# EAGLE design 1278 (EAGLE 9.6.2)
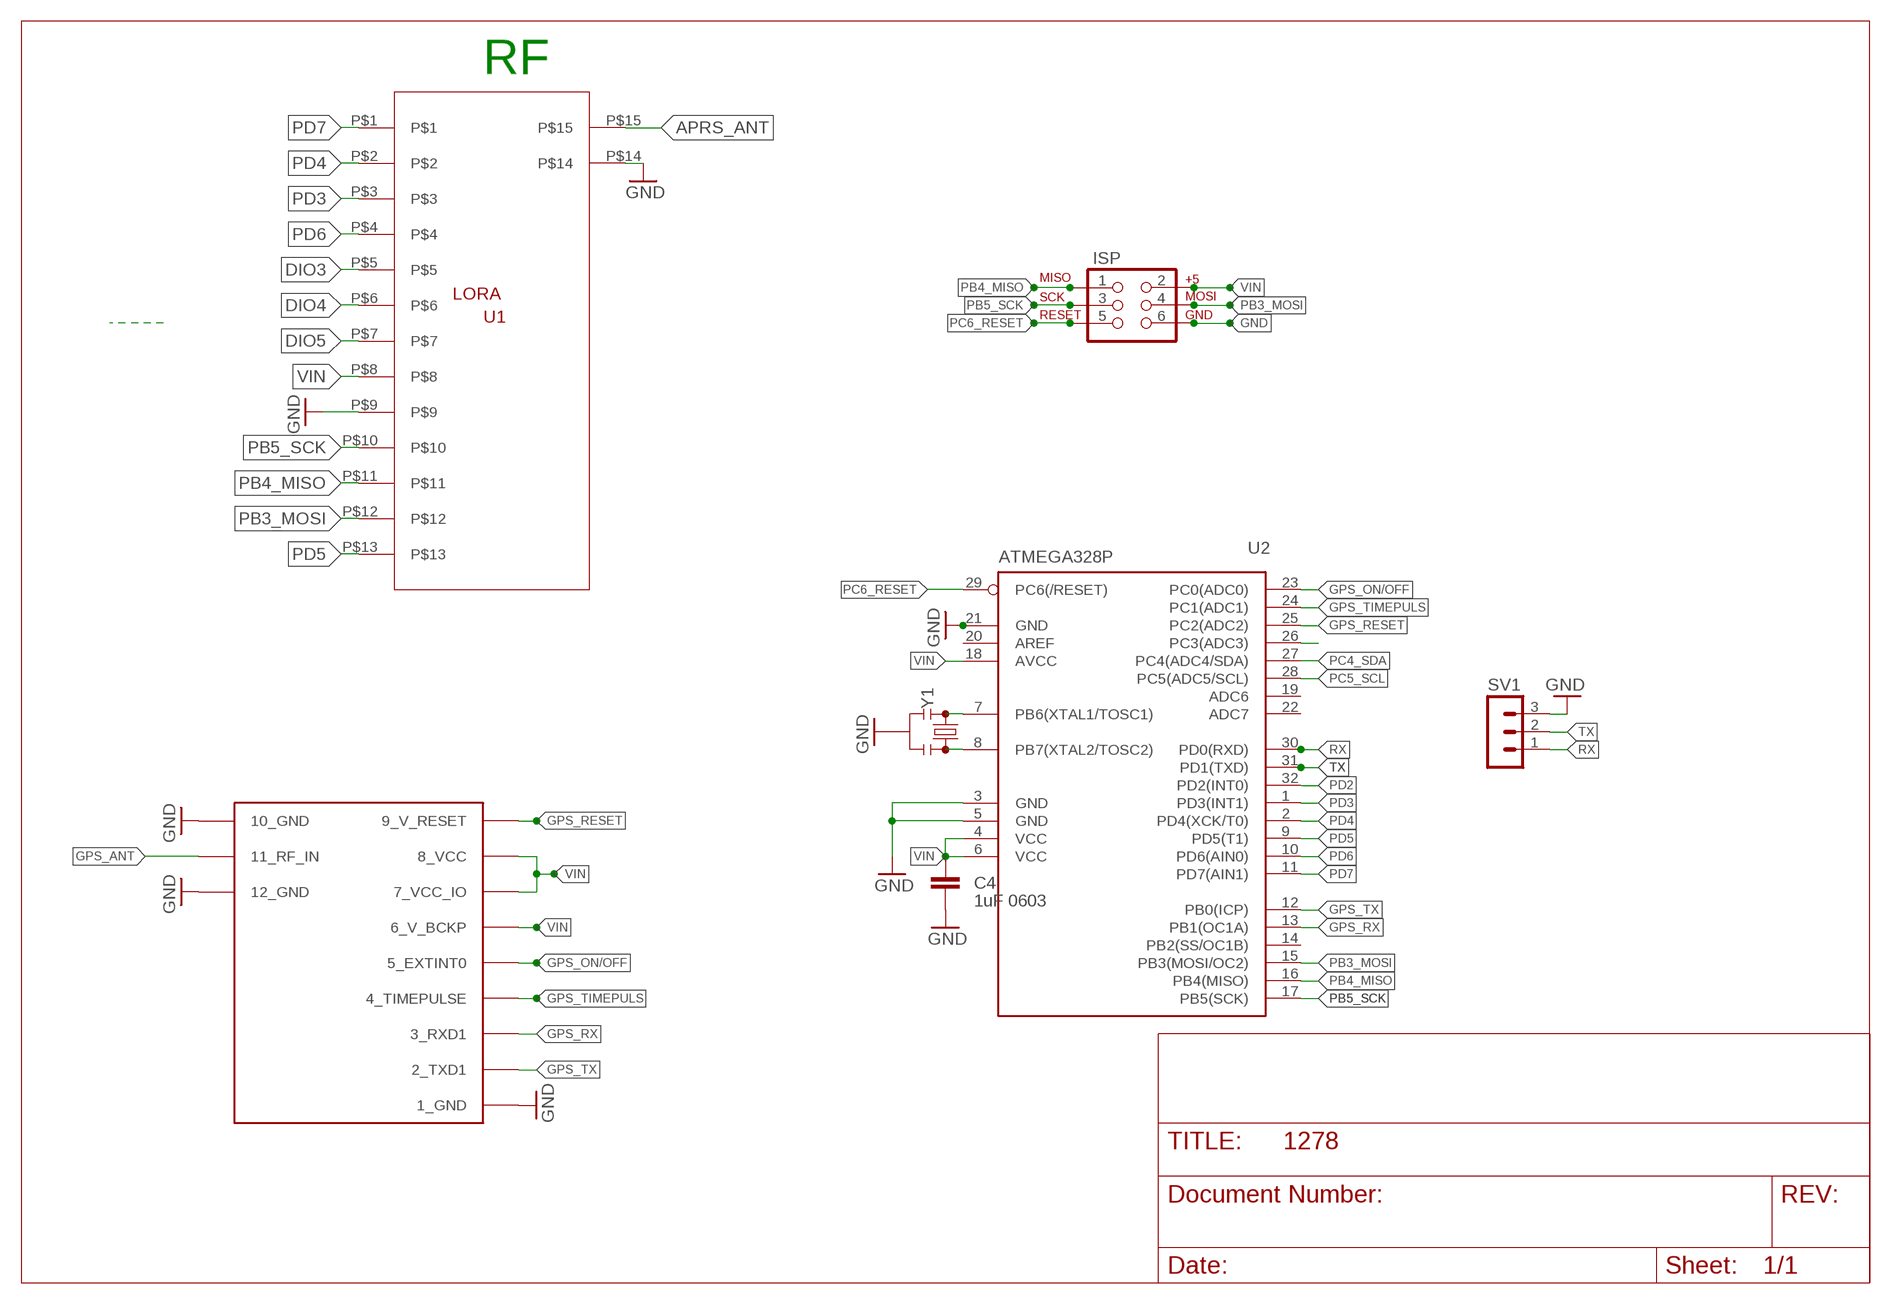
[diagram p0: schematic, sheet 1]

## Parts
C4  1uF 0603  C-EUC0603K  [C0603K]
ISP  AVR_SPI_PRG_6PTH  [2X3]
SV1  MA03-1  [MA03-1]
U1  LORA  [LORA_DRF]
U2  ATMEGA328P  MEGA8-AI  [TQFP32-08]
U$2  UBLOX_MAX  [UBLOX_MAX]
Y1  RESONATORSMD-4.5X2.0  [RESONATOR-SMD-4.5X2.0]

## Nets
APRS_ANT: U1.P$15
DIO3: U1.P$5
DIO4: U1.P$6
DIO5: U1.P$7
GND: C4.2 ISP.6 SV1.3 U1.P$9 U1.P$14 U2.3(GND) U2.5(GND) U2.21(GND) U$2.1_GND U$2.10_GND U$2.12_GND Y1.2
GPS_ANT: U$2.11_RF_IN
GPS_ON/OFF: U2.23(PC0(ADC0)) U$2.5_EXTINT0
GPS_RESET: U2.25(PC2(ADC2)) U$2.9_V_RESET
GPS_RX: U2.13(PB1(OC1A)) U$2.3_RXD1
GPS_TIMEPULS: U2.24(PC1(ADC1)) U$2.4_TIMEPULSE
GPS_TX: U2.12(PB0(ICP)) U$2.2_TXD1
N$1: U2.8(PB7(XTAL2/TOSC2)) Y1.3
N$2: U2.7(PB6(XTAL1/TOSC1)) Y1.1
N$10: U2.26(PC3(ADC3))
PB3_MOSI: ISP.4 U1.P$12 U2.15(PB3(MOSI/OC2))
PB4_MISO: ISP.1 U1.P$11 U2.16(PB4(MISO))
PB5_SCK: ISP.3 U1.P$10 U2.17(PB5(SCK))
PC4_SDA: U2.27(PC4(ADC4/SDA))
PC5_SCL: U2.28(PC5(ADC5/SCL))
PC6_RESET: ISP.5 U2.29(PC6(/RESET))
PD2: U2.32(PD2(INT0))
PD3: U1.P$3 U2.1(PD3(INT1))
PD4: U1.P$2 U2.2(PD4(XCK/T0))
PD5: U1.P$13 U2.9(PD5(T1))
PD6: U1.P$4 U2.10(PD6(AIN0))
PD7: U1.P$1 U2.11(PD7(AIN1))
RX: SV1.1 U2.30(PD0(RXD))
TX: SV1.2 U2.31(PD1(TXD))
VIN: C4.1 ISP.2 U1.P$8 U2.4(VCC) U2.6(VCC) U2.18(AVCC) U$2.6_V_BCKP U$2.7_VCC_IO U$2.8_VCC
Unconnected: U2.14(PB2(SS/OC1B)) U2.19(ADC6) U2.20(AREF) U2.22(ADC7)

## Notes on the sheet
- RF

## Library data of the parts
C4 = rcl:C-EU: CAPACITOR, European symbol; SPICEPREFIX: C
ISP = SparkFun:AVR_SPI_PRG_6: AVR ISP 6 Pin This is the reduced ISP connector for AVR programming. Common on Arduino. This footprint will take up less PCB space and can be used with a 10-pin to 6-pin adapter such as SKU: BOB-08508
SV1 = con-lstb:MA03-1: PIN HEADER; OC_FARNELL: unknown; OC_NEWARK: unknown
U1 = lora:LORA
U2 = atmel:MEGA8: MICROCONTROLLER 8 Kbytes FLASH, 1 kbytes SRAM, 512 bytes EEPROM, USART, 6-channel 10 bit ADC, 2-channel 8 bit ADC Pin compatible with Atmega48, ATMega88, ATMega168 Source: avr.lbr; MPN: ATMEGA8-16AU; OC_FARNELL: 9171371; OC_NEWARK: 73M8863
U$2 = Max gps:UBLOX_MAX: UBLOX MAX
Y1 = SparkFun-Clocks:RESONATOR: Resonators (Generic) Ceramic resonators are clock-generating components, often used to control timing in microcontrollers. They usually have 3 pins: two pins for oscillation, and one pin for ground. Compared to crystals, resonators have worse tolerance, but are usually much cheaper. Plus, they have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

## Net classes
0 default: width 0.152 mm, drill 0.305 mm, clearance 0.152 mm
1 vcc: width 0.152 mm, clearance 0.152 mm

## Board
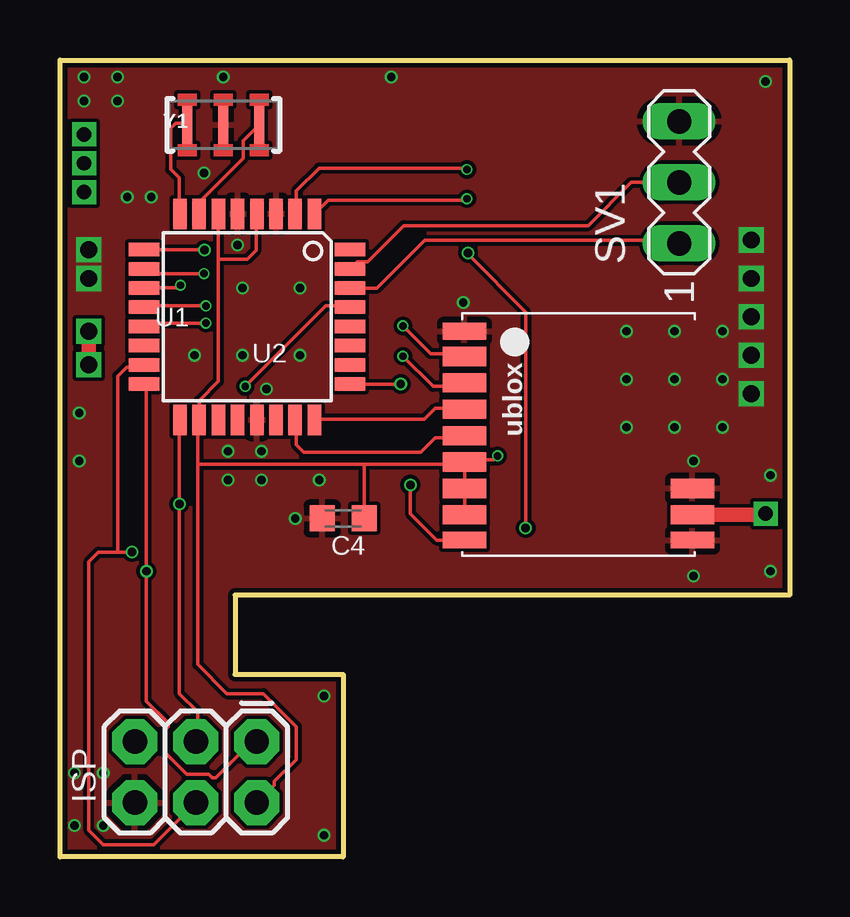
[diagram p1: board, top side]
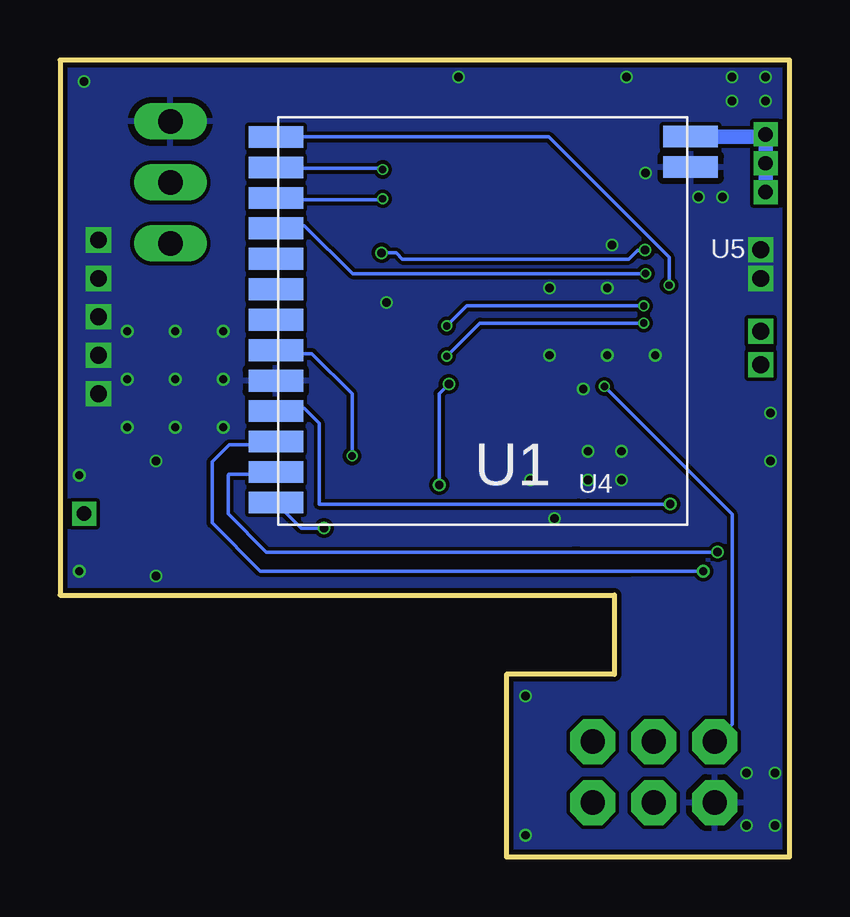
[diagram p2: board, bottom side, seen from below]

Size 30.4 x 33.2 mm. Coordinates in mm from the lower left corner, seen from the top.
Outline: 0,33.2 30.4,33.2 30.4,10.9 7.3,10.9 7.3,7.6 11.8,7.6 11.8,0 0,0 0,33.2
Copper layers (1*16): Top 0.035559375mm / dielectric 1.6mm / Bottom 0.035559375mm
Design rules "jlcpcb2layer *": minimum track width 5mil, minimum drill 12mil, track to track 5mil, track to pad 5mil, pad to pad 5mil, via to via 5mil, smd to smd 5mil, copper to edge 8mil, drill to drill 6mil, minimum pad ring 5mil, minimum via ring 3mil, stop-mask expansion 2.5mil, vias tented up to drill 14mil, thermal gap 10mil

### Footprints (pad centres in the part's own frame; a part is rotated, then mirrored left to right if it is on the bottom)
C0603K = smd 1.05 x 1.08: 1 -0.875,0; 2 0.875,0
2X3 = drill 1.016 pad 1.88 octagon: 1 0,0; 2 0,2.54; 3 2.54,0; 4 2.54,2.54; 5 5.08,0; 6 5.08,2.54
MA03-1 = drill 1.016 long: 1 -2.54,0; 2 0,0; 3 2.54,0
LORA_DRF = smd 2.27 x 0.9: P$1 -8.609,7.497; P$2 -8.609,6.227; P$3 -8.608,4.958; P$4 -8.608,3.688; P$5 -8.609,2.417; P$6 -8.609,1.147; P$7 -8.608,-0.122; P$8 -8.608,-1.392; P$9 -8.61,-2.663; P$10 -8.61,-3.933; P$11 -8.609,-5.202; P$12 -8.609,-6.472; P$13 -8.609,-7.743; P$14 8.673,6.235; P$15 8.675,7.506
TQFP32-08 = smd 1.27 x 0.559: 1 -4.293,2.8; 2 -4.293,2; 3 -4.293,1.2; 4 -4.293,0.4; 5 -4.293,-0.4; 6 -4.293,-1.2; 7 -4.293,-2; 8 -4.293,-2.8; 17 4.293,-2.8; 18 4.293,-2; 19 4.293,-1.2; 20 4.293,-0.4; 21 4.293,0.4; 22 4.293,1.2; 23 4.293,2; 24 4.293,2.8 | smd 0.559 x 1.27: 9 -2.8,-4.293; 10 -2,-4.293; 11 -1.2,-4.293; 12 -0.4,-4.293; 13 0.4,-4.293; 14 1.2,-4.293; 15 2,-4.293; 16 2.8,-4.293; 25 2.8,4.293; 26 2,4.293; 27 1.2,4.293; 28 0.4,4.293; 29 -0.4,4.293; 30 -1.2,4.293; 31 -2,4.293; 32 -2.8,4.293
UBLOX_MAX = smd 1.8 x 0.7: 1_GND 4.95,-4.4; 9_V_RESET 4.95,4.3; 10_GND -4.55,4.3 | smd 1.8 x 0.8: 2_TXD1 4.95,-3.35; 3_RXD1 4.95,-2.25; 4_TIMEPULSE 4.95,-1.15; 5_EXTINT0 4.95,-0.05; 6_V_BCKP 4.95,1.05; 7_VCC_IO 4.95,2.15; 8_VCC 4.95,3.25; 11_RF_IN -4.55,3.25; 12_GND -4.55,2.15
RESONATOR-SMD-4.5X2.0 = smd 0.4 x 1.6: 1 -1.5,0; 2 0,0; 3 1.5,0

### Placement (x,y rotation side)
C4  11.8,14.1 180 top
ISP  8.2,4.8 180 top
SV1  25.8,28.1 90 top
U1  12.8,22.5 0 bottom
U2  7.8,22.5 270 top
U$2  21.8,17.5 180 top
Y1  6.8,30.5 180 top

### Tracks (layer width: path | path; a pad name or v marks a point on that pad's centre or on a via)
APRS_ANT  (via drill 0.6 pad 1)
  Bottom 0.61: U1.P$15 1.09,30.01 v1,30.1 v1,28.9 v1,27.7
GND  (via drill 0.35, 0.7 pad 1)
  Top 0.152: U2.5 7.41,26.76 7.44,26.83
  other vias: 2.8,27.5 13.8,32.5 23.6,19.9 26.4,11.7 7.6,20.9 10.8,15.7 9.8,14.1 0.8,18.5 26.4,16.5 16.8,23.1 10,20.9 8.6,19.5 6.8,32.5 7.4,25.5 6,28.5 3.8,27.5 8.4,16.9 7,16.9 7,15.7 8.4,15.7 7.6,23.7 10,23.7 1.2,24.1 1.2,25.3 28.8,25.7 28.8,24.1 28.8,22.5 28.8,20.9 28.8,19.3 23.6,21.9 25.6,21.9 27.6,21.9 27.6,19.9 25.6,19.9 25.6,17.9 27.6,17.9 23.6,17.9 29.6,15.9 29.6,11.9 5.6,20.9 0.8,16.5 1.8,3.5 11,6.7 11,0.9 1.8,1.3 0.6,3.5 0.6,1.3 29.4,32.3 1,32.5 2.4,32.5 1,31.5 2.4,31.5
  pour Top: -4.59,41.22 49.35,41.22 49.35,-1.89 -4.59,-1.89
  pour Bottom: -4.59,41.22 49.35,41.22 49.35,-1.89 -4.59,-1.89
GPS_ANT  (via drill 0.6 pad 1)
  Top 0.152: 29.35,14.25 v29.4,14.3
  Top 0.61: U$2.11_RF_IN 29.35,14.25
GPS_ON/OFF
  Top 0.152: 16.71,17.46 16.74,17.46 16.84,17.56 | 16.71,17.46 15.64,17.46 15.03,16.86 10.16,16.86 9.85,17.16 9.85,18.07 9.82,18.21 9.85,18.23 U2.23 | 16.71,17.46 U$2.5_EXTINT0
GPS_RESET  (via drill 0.35)
  Top 0.152: U2.25 12.14,19.75 U2.25 v14.2,19.7 | v14.6,15.5 14.6,14.3 15.7,13.2 U$2.9_V_RESET
  Bottom 0.152: v14.2,19.7 14.6,19.3 v14.6,15.5
GPS_RX  (via drill 0.3)
  Top 0.152: v6.08,22.24 3.64,22.24 U2.13 3.6,22.04 3.59,22.04 U2.13 | v14.29,20.86 15.55,19.6 16.7,19.6 | 16.7,19.6 U$2.3_RXD1 | 16.7,19.6 16.71,19.6 U$2.3_RXD1
  Bottom 0.152: v6.08,22.24 12.91,22.24 v14.29,20.86
GPS_TIMEPULS
  Top 0.152: 16.71,18.68 15.64,18.68 15.18,18.23 10.62,18.23 10.61,18.23 | 10.61,18.23 U2.24 | 16.71,18.68 16.85,18.67 | U2.24 10.61,18.23 | 16.71,18.68 U$2.4_TIMEPULSE
GPS_TX  (via drill 0.3)
  Top 0.152: v6.08,22.95 3.6,22.95 | v14.29,22.12 15.44,20.97 16.71,20.97 | 16.71,20.97 16.72,20.97 U$2.2_TXD1 | 3.52,22.89 3.58,22.95 3.6,22.95 | 3.6,22.95 U2.12 | 16.71,20.97 U$2.2_TXD1
  Bottom 0.152: v6.08,22.95 13.46,22.95 v14.29,22.12
N$1
  Top 0.152: 5.28,30.57 5.29,30.57 Y1.3 | 5.28,30.57 4.82,30.57 4.61,30.36 4.61,28.65 4.97,28.29 4.97,26.91 4.99,26.79 4.97,26.76 U2.8 | 5.28,30.57 Y1.3
N$2
  Top 0.152: Y1.1 7.63,29.83 7.63,29.11 5.74,27.21 5.74,26.89 5.81,26.81 U2.7
N$7  (via drill 0.7 pad 1)
  Top 0.61: v1.2,21.9 v1.2,20.5
PB3_MOSI  (via drill 0.35)
  Top 0.152: U2.15 3.45,20.51 3.5,20.51 U2.15 3.42,20.41 2.78,20.41 2.4,20.03 2.4,12.7 | 2.4,12.7 1.6,12.7 1.2,12.3 1.2,1.1 1.8,0.5 3.9,0.5 ISP.4 | 2.4,12.7 v3,12.7
  Bottom 0.152: U1.P$12 21.43,15.94 23.36,15.94 23.4,15.9 23.4,14.3 21.8,12.7 9,12.7 8.8,12.7 v3,12.7
PB4_MISO  (via drill 0.35)
  Top 0.152: v3.6,11.9 3.6,6.49 4.52,5.58 4.52,5.42 4.36,5.27 4.36,4.36 5.28,3.44 6.19,3.44 6.35,3.29 6.5,3.29 7.87,4.66 8.17,4.66 ISP.1 | v3.6,11.9 3.6,19.6 | 3.6,19.6 U2.16 | 3.6,19.6 U2.16 | v3.6,11.9
  Bottom 0.152: U1.P$11 21.41,17.16 23.36,17.16 24.06,16.45 24.06,13.91 22.05,11.9 6.6,11.9 6.2,11.9 v3.6,11.9
PB5_SCK  (via drill 0.35)
  Top 0.152: ISP.3 5.74,4.82 5.74,6.03 4.97,6.8 v4.97,14.7 4.97,18.07 4.99,18.21 4.97,18.23 U2.17
  Bottom 0.152: U1.P$10 21.28,18.68 20.21,18.68 19.6,18.07 19.6,14.7 8.8,14.7 8.4,14.7 v4.97,14.7
PC6_RESET  (via drill 0.3)
  Top 0.152: 11.98,22.95 11.07,22.95 v7.72,19.6 | 11.98,22.95 12.01,22.95 12.08,22.89 | 11.98,22.95 U2.29
  Bottom 0.152: ISP.5 2.4,5.52 2.4,14.28 v7.72,19.6
PD3  (via drill 0.3)
  Top 0.152: v16.96,27.42 16.9,27.36 11.17,27.36 U2.1 10.61,26.76 U2.1
  Bottom 0.152: v16.96,27.42 17,27.37 21.28,27.37 U1.P$3
PD4  (via drill 0.3)
  Top 0.152: 9.85,26.91 9.85,27.75 10.8,28.7 16.89,28.7 v16.96,28.64 | 9.78,26.81 9.85,26.88 9.85,26.91 | 9.85,26.91 U2.2
  Bottom 0.152: v16.96,28.64 17.02,28.7 21.38,28.7 U1.P$2
PD5  (via drill 0.35)
  Top 0.152: v19.4,13.7 19.4,22.7 17,25.1 v17,25.17 | U2.9 6,25.3 v6.02,25.28
  Bottom 0.152: U1.P$13 20.35,13.7 v19.4,13.7 | v6.02,25.28 6.32,25.28 6.71,24.9 16.13,24.9 16.4,25.17 v17,25.17
PD6  (via drill 0.3)
  Top 0.152: 3.51,24.49 3.6,24.48 U2.10 3.71,24.3 v6,24.3
  Bottom 0.152: v6,24.3 18.21,24.3 20.21,26.3 21.28,26.3 U1.P$4
PD7  (via drill 0.3)
  Top 0.152: 3.6,23.71 4.92,23.71 v5.02,23.82 | 3.6,23.71 U2.11 | 3.6,23.71 U2.11
  Bottom 0.152: v5.02,23.82 5.02,24.98 9.67,29.63 9.77,29.73 9.97,29.93 10.04,30 U1.P$1 21.28,29.96 21.13,29.81
RX
  Top 0.152: U2.30 13.2,23.7 15.2,25.7 25.66,25.7 SV1.1
TX
  Top 0.152: U2.31 12.39,24.79 12.82,24.79 14.33,26.3 22,26.3 23.8,28.1 SV1.2
VIN  (via drill 0.3)
  Top 0.152: 16.86,15.33 16.86,15.34 U$2.7_VCC_IO | 16.86,15.33 16.86,14.26 | U$2.8_VCC 16.86,14.26 | v18.23,16.7 18.08,16.55 16.86,16.55 | 16.86,16.55 U$2.6_V_BCKP 16.86,16.4 16.86,15.48 U$2.7_VCC_IO 16.86,15.33 | 8.17,26.91 8.18,26.9 | 8.18,26.9 8.19,26.79 | 6.6,24.9 U2.6 6.65,26.76 6.65,26.75 U2.6 | 6.6,24.9 6.6,19.81 5.8,19.01 U2.18 | U2.18 5.74,18.22 5.74,18.23 U2.18 | 8.17,26.76 U2.4 | 5.74,16.35 5.74,18.11 5.82,18.19 5.89,18.23 U2.18 | 5.74,16.35 5.74,8.02 6.95,6.8 8.48,6.8 9.85,5.42 9.85,4.05 8.94,3.14 8.94,2.99 8.33,2.38 ISP.2 | 5.74,16.35 12.6,16.35 | 12.6,16.35 12.68,16.35 16.75,16.35 U$2.6_V_BCKP | U$2.6_V_BCKP 16.73,16.55 16.71,16.55 U$2.6_V_BCKP | 16.86,14.26 U$2.8_VCC | 16.86,15.33 U$2.7_VCC_IO | 16.86,16.55 U$2.6_V_BCKP | 8.17,26.76 U2.4 8.18,26.82 8.18,26.9 | 6.6,24.9 7.8,24.9 8.17,25.27 8.17,26.76 | C4.1 12.68,16.27 12.6,16.35
  Bottom 0.152: v18.23,16.7 18.23,19.29 19.91,20.97 21.28,20.97 U1.P$8

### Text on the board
tNames: U1
bNames: U5 | U4

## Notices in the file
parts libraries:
SparkFun-Clocks: Licensing: Creative Commons ShareAlike 4.0 International - https://creativecommons.org/licenses/by-sa/4.0
